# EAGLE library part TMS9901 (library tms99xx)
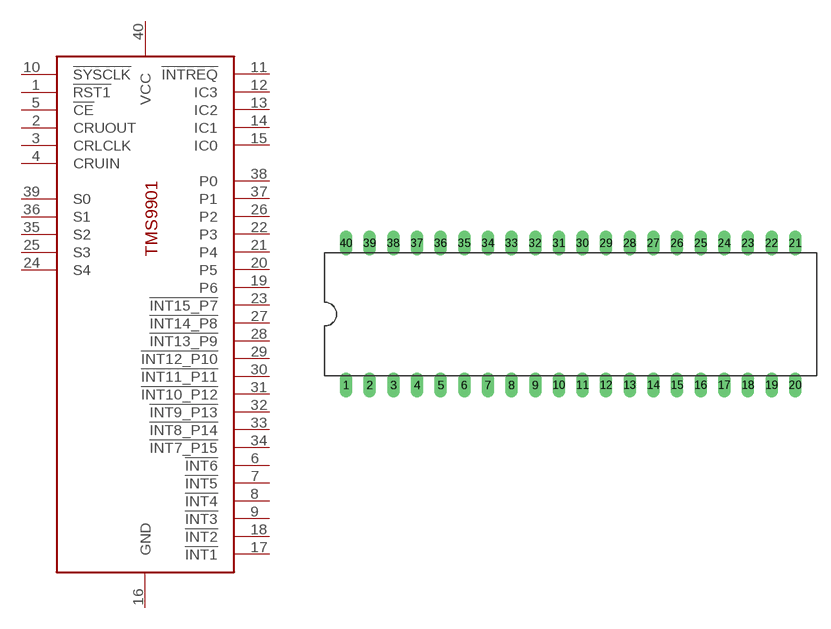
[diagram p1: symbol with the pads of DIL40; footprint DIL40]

Designator prefix -

## TMS9901  [DIL40]
1  !RST1  in
2  CRUOUT  in
3  CRLCLK  in
4  CRUIN  out
5  !CE  in
6  !INT6  in
7  !INT5  in
8  !INT4  in
9  !INT3  in
10  !SYSCLK  in
11  !INTREQ
12  IC3  out
13  IC2  out
14  IC1  out
15  IC0  out
16  GND  pwr
17  !INT1  in
18  !INT2  in
19  P6
20  P5
21  P4
22  P3
23  !INT15_P7
24  S4  in
25  S3  in
26  P2
27  !INT14_P8
28  !INT13_P9
29  !INT12_P10
30  !INT11_P11
31  !INT10_P12
32  !INT9_P13
33  !INT8_P14
34  !INT7_P15
35  S2  in
36  S1  in
37  P1
38  P0
39  S0
40  VCC  pwr

## Footprint DIL40 (pad centres in mm)
Dual In Line
drill 0.813 long: 1 -24.13,-7.62; 2 -21.59,-7.62; 3 -19.05,-7.62; 4 -16.51,-7.62; 5 -13.97,-7.62; 6 -11.43,-7.62; 7 -8.89,-7.62; 8 -6.35,-7.62; 9 -3.81,-7.62; 10 -1.27,-7.62; 11 1.27,-7.62; 12 3.81,-7.62; 13 6.35,-7.62; 14 8.89,-7.62; 15 11.43,-7.62; 16 13.97,-7.62; 17 16.51,-7.62; 18 19.05,-7.62; 19 21.59,-7.62; 20 24.13,-7.62; 21 24.13,7.62; 22 21.59,7.62; 23 19.05,7.62; 24 16.51,7.62; 25 13.97,7.62; 26 11.43,7.62; 27 8.89,7.62; 28 6.35,7.62; 29 3.81,7.62; 30 1.27,7.62; 31 -1.27,7.62; 32 -3.81,7.62; 33 -6.35,7.62; 34 -8.89,7.62; 35 -11.43,7.62; 36 -13.97,7.62; 37 -16.51,7.62; 38 -19.05,7.62; 39 -21.59,7.62; 40 -24.13,7.62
